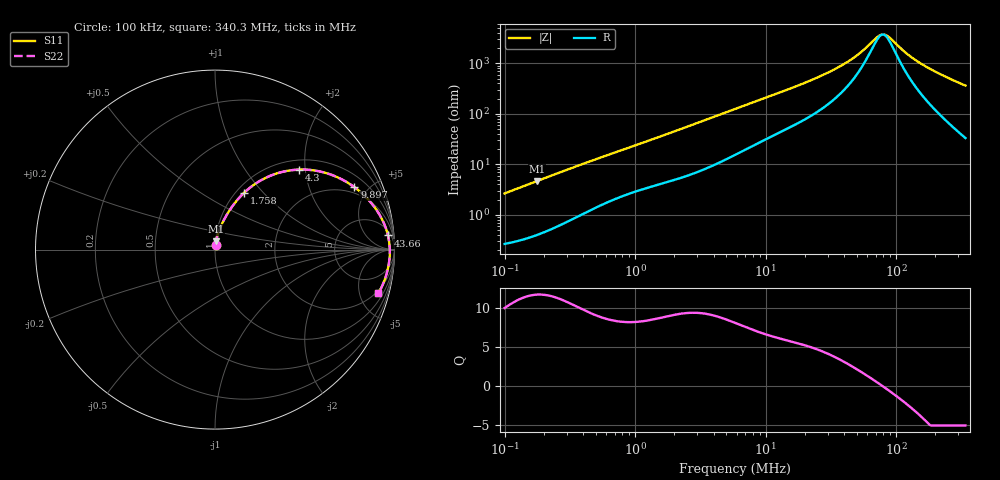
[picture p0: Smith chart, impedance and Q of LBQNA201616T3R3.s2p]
! LBQNA201616T3R3  S-PARAMETER MODEL  ( General Type )
! Model Generated by TAIYO YUDEN Corporation (http://www.ty-top.com)
! Version 1.0
! TAIYO YUDEN Control No. 191025NI43SB-FBB
! Copyright(c) 2019 TAIYO YUDEN CO.,LTD. All Rights Reserved.
! Product Description (link to TY-COMPAS)
! https://ds.yuden.co.jp/TYCOMPAS/or/detail?pn=LBQNA201616T3R3M&u=M
! Products Name : Inductors
! Characteristics :
!  Inductance : 3.3 uH , SRF(min) : 55 MHz , DC Resistance(max) : 0.26 Ohm
!  Rated Current : Saturation :400 mA , Temp Rise : 440 mA (20 degC)
!  Case Size : 2.0 x 1.6 / 0.079 x 0.063 [mm/inch] , Thickness : 1.6 / 0.063 [mm/inch]
!  (Conditions: Temperature = 25 degC , DC Bias Current/Voltage = 0A / 0V)
! External Node Assignments :
!  1  o---GGG---o  2
! GND o---------o GND
! Frequency Range : 0.1MHz  -  340.31115MHz  [ 402 STEP ]
# MHz S RI R 50
! Freq[MHz].  S11 Real  S11 Imag  S21 Real  S21 Imag  S12 Real  S12 Imag  S22 Real  S22 Imag
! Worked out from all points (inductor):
!   401 points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, 100 kHz to 340.3 MHz, reference 50 ohm
!   read as one part in series: L = 4.2 uH near 104.2 kHz
!   highest Q = 11.7 at 176.7 kHz (marker M1), where L = 4.18 uH
!   self-resonance near 79.18 MHz
!   S11 on the Smith chart (normalised r, x): 100 kHz: 1.01, +0.05; 1.758 MHz: 1.09, +0.79; 4.3 MHz: 1.21, +1.85; 9.897 MHz: 1.61, +4.07; 43.66 MHz: 9, +21; 340.3 MHz: 1.66, -7.21
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0.1  0.00334 0.0263  0.9967 -0.0263  0.9967 -0.0263  0.00334 0.0263
0.176698  0.00609 0.046  0.9939 -0.046  0.9939 -0.046  0.00609 0.046
0.390471  0.0196 0.0967  0.9804 -0.0967  0.9804 -0.0967  0.0196 0.0967
0.845508  0.0605 0.185  0.9395 -0.185  0.9395 -0.185  0.0605 0.185
1.524679  0.134 0.2878  0.866 -0.2878  0.866 -0.2878  0.134 0.2878
1.757868  0.1622 0.3167  0.8378 -0.3167  0.8378 -0.3167  0.1622 0.3167
2.639856  0.275 0.3962  0.725 -0.3962  0.725 -0.3962  0.275 0.3962
4.30024  0.4685 0.4458  0.5315 -0.4458  0.5315 -0.4458  0.4685 0.4458
5.953437  0.6053 0.4303  0.3947 -0.4303  0.3947 -0.4303  0.6053 0.4303
9.897147  0.7764 0.3481  0.2236 -0.3481  0.2236 -0.3481  0.7764 0.3481
14.56378  0.8618 0.2699  0.1382 -0.2699  0.1382 -0.2699  0.8618 0.2699
22.77862  0.923 0.1837  0.077 -0.1837  0.077 -0.1837  0.923 0.1837
32.84443  0.9512 0.1215  0.0488 -0.1215  0.0488 -0.1215  0.9512 0.1215
43.65937  0.9638 0.0788  0.0362 -0.0788  0.0362 -0.0788  0.9638 0.0788
53.50253  0.9693 0.0508  0.0307 -0.0508  0.0307 -0.0508  0.9693 0.0508
74.0712  0.9736 0.00851  0.0264 -0.00851  0.0264 -0.00851  0.9736 0.00851
80.34672  0.9739 -0.00188  0.0261 0.00188  0.0261 0.00188  0.9739 -0.00188
88.94399  0.974 -0.0149  0.026 0.0149  0.026 0.0149  0.974 -0.0149
118.2312  0.9719 -0.0527  0.0281 0.0527  0.0281 0.0527  0.9719 -0.0527
153.9991  0.9665 -0.0911  0.0335 0.0911  0.0335 0.0911  0.9665 -0.0911
222.051  0.9505 -0.1534  0.0495 0.1534  0.0495 0.1534  0.9505 -0.1534
340.3111  0.9099 -0.244  0.0901 0.244  0.0901 0.244  0.9099 -0.244
